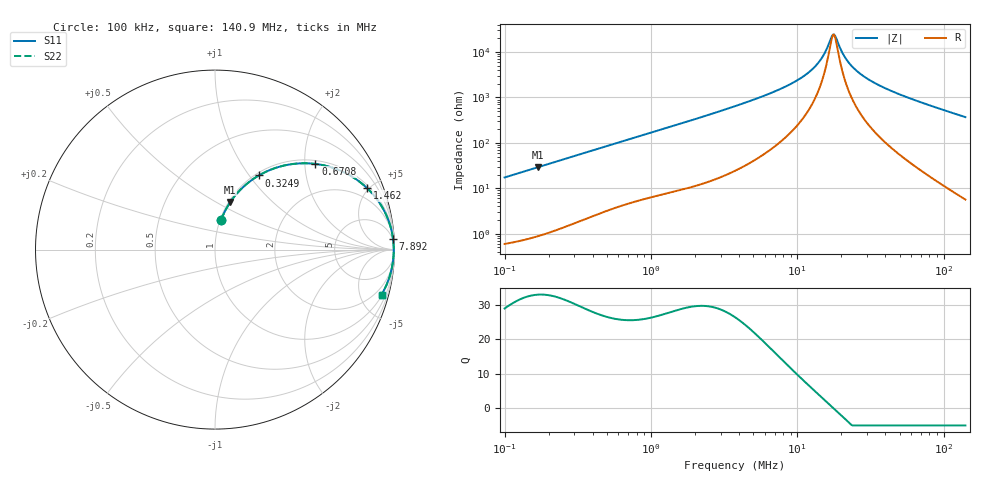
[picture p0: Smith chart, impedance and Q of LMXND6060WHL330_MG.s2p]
! LMXND6060WHL330_MG  S-PARAMETER MODEL  ( General Type )
! Model Generated by TAIYO YUDEN Corporation (http://www.ty-top.com)
! Version 1.0
! TAIYO YUDEN Control No. 191025NI43SB-FBB
! Copyright(c) 2019 TAIYO YUDEN CO.,LTD. All Rights Reserved.
! Product Description (link to TY-COMPAS)
! https://ds.yuden.co.jp/TYCOMPAS/or/detail?pn=LMXND6060WHL330MMG&u=M
! Products Name : Inductors
! Characteristics :
!  Inductance : 33 uH , SRF(min) : 10 MHz , DC Resistance(max) : 0.286 Ohm
!  Rated Current : Saturation :1100 mA , Temp Rise : 1100 mA
!  Case Size : 6.0 x 6.0 / 0.236 x 0.236 [mm/inch] , Thickness : 2.8 / 0.11 [mm/inch]
!  (Conditions: Temperature = 25 degC , DC Bias Current/Voltage = 0A / 0V)
! External Node Assignments :
!  1  o---GGG---o  2
! GND o---------o GND
! Frequency Range : 0.1MHz  -  140.89697MHz  [ 402 STEP ]
# MHz S RI R 50
! Freq[MHz].  S11 Real  S11 Imag  S21 Real  S21 Imag  S12 Real  S12 Imag  S22 Real  S22 Imag
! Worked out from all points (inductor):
!   401 points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, 100 kHz to 140.9 MHz, reference 50 ohm
!   read as one part in series: L = 27.6 uH near 103.7 kHz
!   highest Q = 33 at 169.2 kHz (marker M1), where L = 27.5 uH
!   self-resonance near 17.52 MHz
!   S11 on the Smith chart (normalised r, x): 100 kHz: 1.01, +0.35; 324.9 kHz: 1.04, +1.11; 670.8 kHz: 1.09, +2.26; 1.462 MHz: 1.17, +4.85; 7.892 MHz: 3, +32; 140.9 MHz: 1.11, -7.38
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0.1  0.0346 0.1664  0.9654 -0.1664  0.9654 -0.1664  0.0346 0.1664
0.169159  0.0856 0.2651  0.9144 -0.2651  0.9144 -0.2651  0.0856 0.2651
0.32486  0.2445 0.4133  0.7555 -0.4133  0.7555 -0.4133  0.2445 0.4133
0.336853  0.2574 0.4205  0.7426 -0.4205  0.7426 -0.4205  0.2574 0.4205
0.67079  0.559 0.4774  0.441 -0.4774  0.441 -0.4774  0.559 0.4774
1.134703  0.7728 0.4008  0.2272 -0.4008  0.2272 -0.4008  0.7728 0.4008
1.462492  0.8465 0.3433  0.1535 -0.3433  0.1535 -0.3433  0.8465 0.3433
3.753625  0.9709 0.1502  0.0291 -0.1502  0.0291 -0.1502  0.9709 0.1502
7.892476  0.9918 0.0614  0.00822 -0.0614  0.00822 -0.0614  0.9918 0.0614
10.3585  0.9943 0.0385  0.00573 -0.0385  0.00573 -0.0385  0.9943 0.0385
12.64421  0.9953 0.0235  0.00471 -0.0235  0.00471 -0.0235  0.9953 0.0235
14.61739  0.9957 0.0132  0.00428 -0.0132  0.00428 -0.0132  0.9957 0.0132
15.71661  0.9958 0.00821  0.00416 -0.00821  0.00416 -0.00821  0.9958 0.00821
17.2076  0.9959 0.00197  0.00408 -0.00197  0.00408 -0.00197  0.9959 0.00197
17.84287  0.9959 -0.000515  0.00407 0.000515  0.00407 0.000515  0.9959 -0.000515
18.5016  0.9959 -0.003  0.00407 0.003  0.00407 0.003  0.9959 -0.003
21.00463  0.9958 -0.0118  0.00418 0.0118  0.00418 0.0118  0.9958 -0.0118
24.28248  0.9955 -0.022  0.00452 0.022  0.00452 0.022  0.9955 -0.022
30.73494  0.9944 -0.0397  0.0056 0.0397  0.0056 0.0397  0.9944 -0.0397
42.59248  0.9913 -0.068  0.00867 0.068  0.00867 0.068  0.9913 -0.068
72.04905  0.979 -0.129  0.021 0.129  0.021 0.129  0.979 -0.129
140.897  0.9283 -0.2505  0.0717 0.2505  0.0717 0.2505  0.9283 -0.2505
